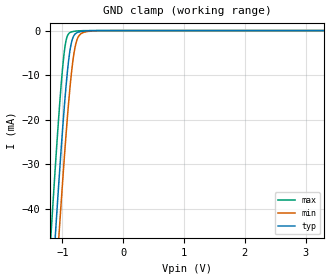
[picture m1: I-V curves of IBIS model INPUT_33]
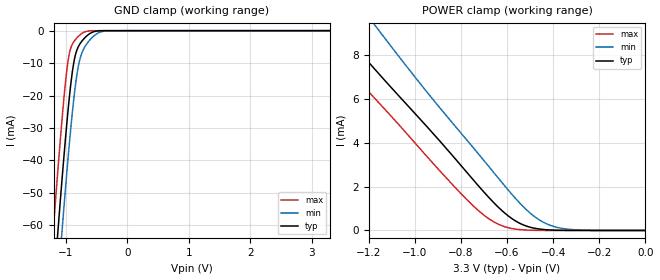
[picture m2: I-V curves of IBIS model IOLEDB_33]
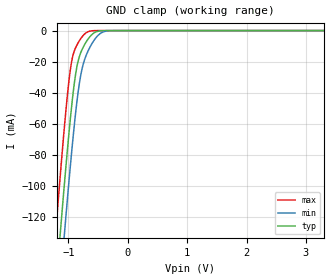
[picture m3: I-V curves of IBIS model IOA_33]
| TEXAS INSTRUMENTS INCORPORATED
| Standard Linear and Logic Group
| IBIS Model of TS3DV20812
| 2-Gbps Differential Switch 8-Bits, 1: 2 MUX/DEMUX With 3-Side Band Signals
| This file contains package information for the following:
|  QFN 36-pin (RHH) package as [Component] TS3DV20812RHH
| This device can be powered at the following Vccs:
|  3.3 volt Vcc
| This file provides unique models under the [Model Selector] for each Vcc.
| For operation at a specific Vcc, select the appropriate model after each
| [Model Selector] keyword.
[IBIS Ver]   3.2
[Comment char]  |_char
[File Name]   ts3dv20812.ibs
[File Rev]   1.2 | x_die
[Date]   January 24, 2012
[Source]   Data created from TI-SPICE simulations at TI-SLL.
[Notes]   The following is an IBIS list for the SN74TS3DV20812.
   Please contact sllibis@ti.com with questions and
   comments concerning SLL IBIS models.
   - FILE REV HISTORY
   - 1.1 Release IBIS file on 11/05/08
   - Power clamp data deleted was deleted as there is no
   power-clamp diode.
   - Non-monotonic data due to FET characteristics.
   - 1.2 Release TS3DV20812 based on TS3L4892 IBIS model on 1/24/12
[Disclaimer] Property of Texas Instruments Incorporated.  Unauthorized
   reproduction and/or distribution is strictly prohibited.
   This product is protected under copyright law.
   Created  2012, (C) Copyright  2012, Texas Instruments
   Incorporated, All Rights Reserved
   UNLESS THERE IS A SIGNED, WRITTEN AGREEMENT TO THE
   CONTRARY, TEXAS INSTRUMENTS (TI) IS PROVIDING THE IBIS
   MODELS  AND WITHOUT ANY WARRANTY, EXPRESSED OR
   IMPLIED.  TI assumes no liability for:
   1) the accuracy of the IBIS models provided to your
   company;
   2) the proper functioning of these IBIS Models in your
   design or for any resulting applications; or
   3) infringement of patents, copyrights or intellectual
   property rights resulting from your use of these IBIS
   models.
   TI provides IBIS Models as a service to our customers.
   You and your company shall not distribute, sell or give
   these models to anyone else without prior written
   permission from TI.
   TI reserves the right to make changes to our products or
   to discontinue any semiconductor product or service
   without notice, and advises our customers to obtain the
   latest version of relevant information to verify, before
   placing orders, that the information being relied on is
   current.
   Please be aware that your receipt and use of the IBIS
   information provided shall serve as acceptance of these
   terms and conditions.  If you do not accept these terms,
   you should return or destroy the IBIS models and any
   other accompanying information immediately.
| Component TS3DV20812RHH 36-PIN QFN
[Component]   TS3DV20812RHH
[Manufacturer]   Texas Instruments, Inc.
[Package]
|   typ   min   max
R_pkg   7.800e-02   1.000e-03   9.600e-02
L_pkg   2.086e-09   1.110e-10   2.529e-09
C_pkg   2.440e-13   9.400e-14   2.970e-13
[Pin]   signal_name   model_name   R_pin   L_pin   C_pin
1   1A   IOA_33   9.500e-02   2.497e-09   2.640e-13
2   2A   IOA_33   8.900e-02   2.321e-09   2.220e-13
3   3A   IOA_33   8.400e-02   2.255e-09   2.740e-13
4   0LED   IOLEDA_33   8.100e-02   2.179e-09   2.570e-13
5   0LED1   IOLEDB_33   7.900e-02   2.060e-09   1.980e-13
6   0LED2   IOLEDB_33   8.100e-02   2.179e-09   2.570e-13
7   4A   IOA_33   8.400e-02   2.255e-09   2.740e-13
8   5A   IOA_33   8.900e-02   2.321e-09   2.220e-13
9   6A   IOA_33   9.500e-02   2.497e-09   2.610e-13
10   7A   IOA_33   9.100e-02   2.420e-09   2.740e-13
11   GND   GND   7.400e-02   1.965e-09   2.250e-13
12   1LED   IOLEDA_33   6.900e-02   1.828e-09   2.160e-13
13   1LED1   IOLEDB_33   6.600e-02   1.839e-09   2.780e-13
14   1LED2   IOLEDB_33   6.300e-02   1.682e-09   1.990e-13
15   7B2   IOB_33   6.600e-02   1.845e-09   2.790e-13
16   6B2   IOB_33   6.900e-02   1.839e-09   2.160e-13
17   7B1   IOB_33   7.600e-02   2.013e-09   2.270e-13
18   6B1   IOB_33   8.600e-02   2.311e-09   2.690e-13
19   5B2   IOB_33   9.600e-02   2.529e-09   2.560e-13
20   4B2   IOB_33   9.000e-02   2.350e-09   2.220e-13
21   5B1   IOB_33   8.500e-02   2.279e-09   2.740e-13
22   4B1   IOB_33   8.200e-02   2.197e-09   2.570e-13
23   3B2   IOB_33   7.900e-02   2.071e-09   1.970e-13
24   2B2   IOB_33   8.100e-02   2.181e-09   2.560e-13
25   3B1   IOB_33   8.400e-02   2.248e-09   2.720e-13
26   2B1   IOB_33   8.800e-02   2.307e-09   2.190e-13
27   SEL   INPUT_33   8.900e-02   2.348e-09   2.510e-13
28   1B2   IOB_33   8.500e-02   2.293e-09   2.810e-13
29   0B2   IOB_33   7.600e-02   2.012e-09   2.340e-13
30   1B1   IOB_33   6.900e-02   1.839e-09   2.180e-13
31   0B1   IOB_33   6.600e-02   1.845e-09   2.940e-13
32   2LED2   IOLEDB_33   1.000e-03   1.110e-10   9.400e-14
33   2LED1   IOLEDB_33   6.600e-02   1.839e-09   2.940e-13
34   2LED   IOLEDA_33   6.900e-02   1.828e-09   2.180e-13
35   VCC   POWER   7.800e-02   2.073e-09   2.400e-13
36   0A   IOA_33   9.100e-02   2.445e-09   2.970e-13
[Series Switch Groups]
| Function Group States
On  1 /   | 0A-7A->0B1-7B1 SEL1 LOW
   | 0B1-7B1->0A-7A SEL1 LOW
On  2 /   | 0LED->0LED1 SEL1 LOW
   | 0LED1->0LED SEL1 LOW
On  3 /   | 1LED->1LED1 SEL2 LOW
   | 1LED1->1LED SEL2 LOW
On  4 /   | 2LED->2LED1 SEL2 LOW
   | 2LED1->2LED SEL2 LOW
On  5 /   | 0A-7A->0B2-7B2 SEL1 HIGH
   | 0B2-7B2->0A-7A SEL1 HIGH
On  6 /   | 0LED->0LED2 SEL1 HIGH
   | 0LED2->0LED SEL1 HIGH
On  7 /   | 1LED->1LED2 SEL1 HIGH
   | 1LED2->1LED SEL1 HIGH
On  8 /   | 2LED->2LED2 SEL1 HIGH
   | 2LED2->2LED SEL1 HIGH
[Series Pin Mapping]   pin_2   model_name   function_table_group
36   31   IOA_33_S   1
1   30   IOA_33_S   1
2   26   IOA_33_S   1
3   25   IOA_33_S   1
7   22   IOA_33_S   1
8   21   IOA_33_S   1
9   18   IOA_33_S   1
10   17   IOA_33_S   1
31   36   IOB_33_S   1
30   1   IOB_33_S   1
26   2   IOB_33_S   1
25   3   IOB_33_S   1
22   7   IOB_33_S   1
21   8   IOB_33_S   1
18   9   IOB_33_S   1
17   10   IOB_33_S   1
4   5   IOLEDA_33_S   2
5   4   IOLEDB_33_S   2
12   13   IOLEDA_33_S   3
13   12   IOLEDB_33_S   3
34   33   IOLEDA_33_S   4
33   34   IOLEDB_33_S   4
36   29   IOA_33_S   5
1   28   IOA_33_S   5
2   24   IOA_33_S   5
3   23   IOA_33_S   5
7   20   IOA_33_S   5
8   19   IOA_33_S   5
9   16   IOA_33_S   5
10   15   IOA_33_S   5
29   36   IOB_33_S   5
28   1   IOB_33_S   5
24   2   IOB_33_S   5
23   3   IOB_33_S   5
20   7   IOB_33_S   5
19   8   IOB_33_S   5
16   9   IOB_33_S   5
15   10   IOB_33_S   5
4   6   IOLEDA_33_S   6
6   4   IOLEDB_33_S   6
12   14   IOLEDA_33_S   7
14   12   IOLEDB_33_S   7
34   32   IOLEDA_33_S   8
32   34   IOLEDB_33_S   8
[Model]   IOLEDB_33_S
Model_type  Series_switch
| variable   typ   min   max
C_comp   0   0   0
[Temperature Range]   40   100   -40
| Ambient temperature   25   85   -40
[Voltage range]   3.3   3   3.6
[On]
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[Off]
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[Model]   IOA_33_S
Model_type  Series_switch
| variable   typ   min   max
C_comp   0   0   0
[Temperature Range]   40   100   -40
| Ambient temperature   25   85   -40
[Voltage range]   3.3   3   3.6
[On]
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[Off]
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[Model]   IOLEDA_33_S
Model_type  Series_switch
| variable   typ   min   max
C_comp   0   0   0
[Temperature Range]   40   100   -40
| Ambient temperature   25   85   -40
[Voltage range]   3.3   3   3.6
[On]
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[Off]
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[Model]   IOB_33_S
Model_type  Series_switch
| variable   typ   min   max
C_comp   0   0   0
[Temperature Range]   40   100   -40
| Ambient temperature   25   85   -40
[Voltage range]   3.3   3   3.6
[On]
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[Off]
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| Models and submodels in the file (9): INPUT_33 (Input), IOLEDB_33_S (Series_switch), IOLEDB_33 (Terminator), IOA_33_S (Series_switch), IOA_33 (Terminator), IOLEDA_33_S (Series_switch), IOLEDA_33 (Terminator), IOB_33_S (Series_switch), IOB_33 (Terminator)
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| Model TS3DV20812_INPUT
| Model TS3DV20812_IOLEDB
| Model TS3DV20812_IOLEDB_S
| Model TS3DV20812_IOA
| Model TS3DV20812_IOA_S
| Model TS3DV20812_IOLEDA
| Model TS3DV20812_IOLEDA_S
| Model TS3DV20812_IOB
| Model TS3DV20812_IOB_S
[Model]   INPUT_33
Model_type  Input
Vinl=0.8
Vinh=2.0
| variable   typ   min   max
C_comp   1.09pF   0.73pF   1.33pF
[Temperature Range]   40   100   -40
| Ambient temperature   25   85   -40
[Voltage range]   3.3   3   3.6
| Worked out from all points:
|   GND clamp passes 1 mA (typ) near -0.81 V on its own axis
[GND Clamp]
| TS3DV20812_INPUT_33
|   Voltage   I(typ)   I(min)   I(max)
-3.3V     -559.2mA   -570mA     -546.4mA
-1.2V     -63.91mA   -76.42mA   -48.38mA
-1.18V    -59.55mA   -72.05mA   -44.01mA
-1.11V    -44.57mA   -57.01mA   -29.16mA
-1.05V    -32.27mA   -44.5mA    -17.33mA
-960mV    -15.59mA   -26.89mA   -3.818mA
-920mV    -9.487mA   -19.78mA   -1.266mA
-870mV    -3.981mA   -11.97mA   -406.9uA
-820mV    -1.358mA   -6.004mA   -196.5uA
-770mV    -544.2uA   -2.483mA   -100.9uA
-605mV    -70.11uA   -245.7uA   -5.516uA
3.3V      158.3pA    34.53nA    40.78pA
[Model]   IOLEDB_33
Model_type  Terminator
| variable   typ   min   max
C_comp   2.84pF   2.46pF   3.12pF
| C_tri-state   2.84pF   2.46pF   3.12pF
[Temperature Range]   40   100   -40
| Ambient temperature   25   85   -40
[Voltage range]   3.3   3   3.6
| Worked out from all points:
|   GND clamp passes 1 mA (typ) near -0.62 V on its own axis
|   POWER clamp passes 1 mA (typ) near -0.63 V on its own axis
[GND Clamp]
| TS3DV20812_IOLEDB_33
|   Voltage   I(typ)   I(min)   I(max)
-3.3V     -663.6mA   -677.1mA   -650.2mA
-1.21V    -82.09mA   -98.52mA   -62.97mA
-1.13V    -62.14mA   -78.4mA    -43.15mA
-1.055V   -44.26mA   -60.17mA   -25.87mA
-1V       -31.99mA   -47.38mA   -14.91mA
-950mV    -21.9mA    -36.38mA   -7.762mA
-885mV    -11.54mA   -23.55mA   -3.859mA
-825mV    -6.245mA   -14.2mA    -2.33mA
-710mV    -2.568mA   -5.631mA   -540.7uA
-530mV    -243.9uA   -1.396mA   -4.641uA
-320mV    -1.314uA   -45.58uA   -1.134nA
3.3V      1.422nA    28.92uA    43.28pA
[POWER Clamp]
| TS3DV20812_IOLEDB_33
|   Voltage   I(typ)   I(min)   I(max)
-3.3V     35.58mA    37.81mA    37.34mA
-1.435V   10.55mA    13.14mA    9.175mA
-1.335V   9.329mA    11.67mA    7.927mA
-1.3V     8.903mA    11.17mA    7.507mA
-1.185V   7.515mA    9.557mA    6.176mA
-1.145V   7.041mA    9.003mA    5.72mA
-735mV    2.177mA    3.643mA    1.015mA
-645mV    1.14mA     2.489mA    324.5uA
-560mV    416.1uA    1.43mA     58.24uA
-470mV    82.12uA    554.6uA    5.784uA
-390mV    14.55uA    160.6uA    578.2nA
0V        0A         0A         0A
[Model]   IOA_33
Model_type  Terminator
| variable   typ   min   max
C_comp   6.16pF   5.62pF   6.85pF
| C_tri-state   6.16pF   5.62pF   6.85pF
[Temperature Range]   40   100   -40
| Ambient temperature   25   85   -40
[Voltage range]   3.3   3   3.6
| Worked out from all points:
|   GND clamp passes 1 mA (typ) near -0.54 V on its own axis
[GND Clamp]
| TS3DV20812_IOA_33
|   Voltage   I(typ)   I(min)   I(max)
-3.3V     -1.274A    -1.293A    -1.263A
-1.225V   -172mA     -204.9mA   -134.9mA
-1.2V     -160mA     -192.9mA   -122.8mA
-1.14V    -131.6mA   -164.4mA   -94.38mA
-1.06V    -95.23mA   -127.4mA   -58.74mA
-945mV    -48.41mA   -77.9mA    -19.81mA
-875mV    -27.17mA   -51.7mA    -10.73mA
-805mV    -15.53mA   -31.5mA    -5.901mA
-675mV    -5.775mA   -13.61mA   -846uA
-515mV    -557.5uA   -3.648mA   -8.562uA
-350mV    -9.572uA   -260.6uA   -13.01nA
3.3V      4.272nA    414.7nA    3.367nA
